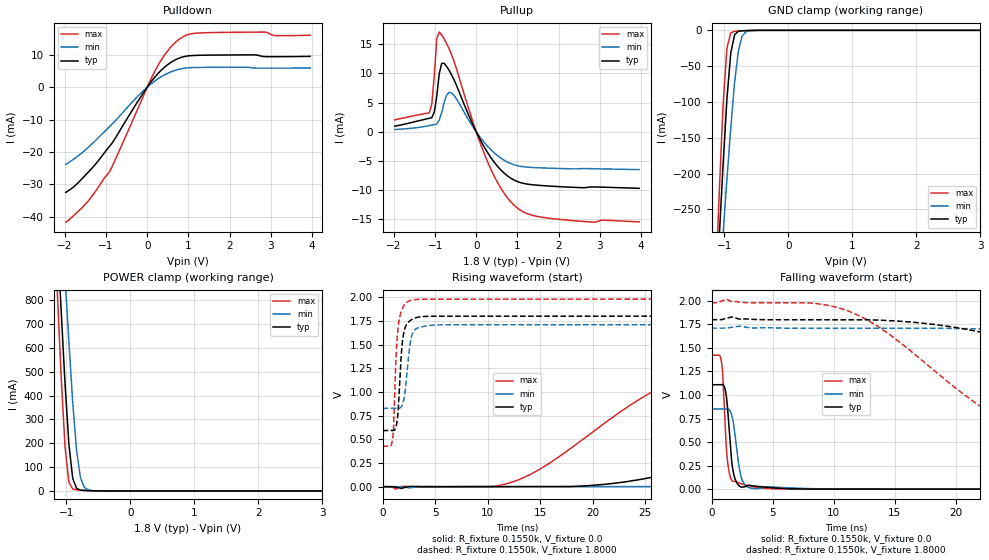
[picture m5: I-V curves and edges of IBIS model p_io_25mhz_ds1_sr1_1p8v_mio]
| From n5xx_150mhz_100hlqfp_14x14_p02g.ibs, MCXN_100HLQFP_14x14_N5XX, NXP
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[Model] p_io_25mhz_ds1_sr1_1p8v_mio
|   Model p_io_25mhz_ds1_sr1_1p8v_mio
| This model was characterised for following simulation conditions:
| External (pad) voltage:
|   - Typ: 1.8V,   - Min: 1.71V,   - Max: 1.98V
| Library cells for typ/min/max conditions are connected as defined below:
|  pad - External Pad
|  ipp_do_lv - Core Input
|  ipp_obe_lv - Output Buffer Enable
|  IOGC - NC
|  REFH3V3 - REFH3V3
|  REFL3V3 - REFL3V3
|  ZI - NC
|  abut_ncal_vddio[1] - vssio vddio vddio
|  abut_ncal_vddio[2] - vddio vddio vssio
|  abut_ncal_vddio[3] - vddio
|  abut_ncal_vddio[4] - vssio vddio vddio
|  abut_ncal_vddio[5] - vddio vddio vssio
|  abut_ncal_vddio[6] - vddio
|  abut_pcal_vddio[1] - vssio
|  abut_pcal_vddio[2] - vddio vssio vddio
|  abut_pcal_vddio[3] - vssio
|  abut_pcal_vddio[4] - vssio
|  abut_pcal_vddio[5] - vddio vssio vddio
|  abut_pcal_vddio[6] - vssio
|  ipp_do_1p8v - ipp_do_1p8v
|  ipp_dse_lv - vdd_lv
|  ipp_eftd_lv - NC
|  ipp_ina_mux_vddio - NC
|  ipp_ina_mux_vddio[0] - NC
|  ipp_ina_mux_vddio[1] - NC
|  ipp_ina_r0_vddio - NC
|  ipp_ina_r0a_vddio - NC
|  ipp_ina_r0b_vddio - NC
|  ipp_ina_r0c_vddio - NC
|  ipp_ina_r0d_vddio - NC
|  ipp_ina_r0e_vddio - NC
|  ipp_ina_r0f_vddio - NC
|  ipp_ina_r300_vddio - NC
|  ipp_ina_r300a_vddio - NC
|  ipp_ina_r300b_vddio - NC
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Model_type I/O
Polarity   Non-Inverting
Enable   Active-High
Vinl =   0.5400V
Vinh =   1.2600V
Vmeas =  0.9000V
Cref =   30.0000pF
Rref =   1.0000M
Vref =   1.8000V
C_comp   1.3069pF   1.2545pF   1.3693pF
|C_comp_pullup   0.5684pF   0.5978pF   0.5415pF
|C_comp_pulldown   0.6467pF   0.6779pF   0.6223pF
[Model Spec]
| variable   typ   min   max
Vinh   1.2600V   1.1970V   1.3860V
Vinl   0.5400V   0.5130V   0.5940V
[Temperature Range]   25.0000   0.1250k   -40.0000
[Voltage Range]   1.8000V   1.7100V   1.9800V
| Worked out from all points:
|   slope of the pulldown table from 0 to 0.27 V, typ, clamps not added: 62.4 ohm
|   slope of the pullup table from 0 to 0.27 V, typ, clamps not added: 77.5 ohm
|   GND clamp passes 1 mA (typ) near -0.75 V on its own axis
|   POWER clamp passes 1 mA (typ) near -0.63 V on its own axis
|   rising waveform, R_fixture 0.1550k, V_fixture 0.0: 20-80 % time 23.8ns typ, 44.7ns min, 12ns max; typ from 0 V to 1.11 V
|   rising waveform, R_fixture 0.1550k, V_fixture 1.8000: 20-80 % time 417ps typ, 512ps min, 381ps max; typ from 0.592 V to 1.8 V
|   falling waveform, R_fixture 0.1550k, V_fixture 0.0: 20-80 % time 432ps typ, 534ps min, 371ps max; typ from 1.11 V to 0 V
|   falling waveform, R_fixture 0.1550k, V_fixture 1.8000: 20-80 % time 19.3ns typ, 37.7ns min, 9.58ns max; typ from 1.8 V to 0.592 V
[Pulldown]
|Voltage   I(typ)   I(min)   I(max)
-1.98V    -32.47mA   -23.82mA   -41.66mA
-1.44V    -26.32mA   -18.64mA   -35.17mA
-900mV    -18mA      -11.95mA   -25.72mA
-180mV    -3.436mA   -2.171mA   -5.242mA
180mV     3.037mA    1.878mA    4.808mA
480mV     6.796mA    4.207mA    10.95mA
780mV     8.996mA    5.568mA    14.83mA
1.02V     9.701mA    6.008mA    16.34mA
1.38V     9.88mA     6.118mA    16.8mA
2.88V     9.438mA    5.883mA    17mA
3.12V     9.431mA    5.886mA    15.93mA
3.96V     9.527mA    5.94mA     16.05mA
[Pullup]
|Voltage   I(typ)   I(min)   I(max)
-1.98V    967.4uA    399.6uA    2.046mA
-1.14V    2.322mA    1.064mA    3.245mA
-1.08V    2.417mA    1.15mA     4.767mA
-1.02V    3.36mA     1.241mA    9.562mA
-960mV    6.043mA    1.333mA    15.9mA
-900mV    9.924mA    1.975mA    17.07mA
-780mV    11.72mA    5.036mA    15.9mA
-600mV    9.761mA    6.668mA    13.21mA
240mV     -3.146mA   -2.19mA    -4.535mA
900mV     -8.187mA   -5.593mA   -12.43mA
1.68V     -9.242mA   -6.203mA   -14.71mA
3.96V     -9.672mA   -6.474mA   -15.42mA
[GND_clamp]
|Voltage   I(typ)   I(min)   I(max)
-1.98V    -1.998A    -1.645A    -2.498A
-1.14V    -394mA     -441.4mA   -363.8mA
-1.08V    -288.3mA   -361.7mA   -226.5mA
-1.02V    -187.2mA   -283.6mA   -103.9mA
-960mV    -95.66mA   -207.9mA   -24.8mA
-900mV    -31.51mA   -136.2mA   -3.52mA
-840mV    -6.042mA   -72.18mA   -1.393mA
-780mV    -1.326mA   -27.91mA   -950.1uA
-720mV    -597.6uA   -7.636mA   -651.3uA
-660mV    -360.6uA   -1.814mA   -411.4uA
-420mV    -15.1uA    -32.81uA   -9.558uA
3.96V     0A         0A         0A
[POWER_clamp]
|Voltage   I(typ)   I(min)   I(max)
-1.98V    5.618A     5.349A     6.084A
-1.14V    1.071A     1.443A     829.5mA
-1.08V    754.2mA    1.168A     476.4mA
-1.02V    449mA      895.6mA    184.5mA
-960mV    195.8mA    625.5mA    36.73mA
-900mV    52.41mA    371.1mA    7.756mA
-840mV    10.72mA    170.2mA    4.398mA
-780mV    3.601mA    56.22mA    3.157mA
-720mV    2.062mA    15.03mA    2.179mA
-660mV    1.299mA    4.293mA    1.367mA
-360mV    5.029uA    27.47uA    1.319uA
3.96V     0A         0A         0A
[Ramp]
| variable   typ   min   max
dV/dt_r  0.6653/23.7529n   0.5079/44.7216n   0.8533/12.0054n
dV/dt_f  0.7248/19.2931n   0.5284/37.7240n   0.9320/9.5760n
R_load = 0.1550k
[Rising Waveform]
R_fixture= 0.1550k
V_fixture= 0.0
V_fixture_min= 0.0
V_fixture_max= 0.0
|time   V(typ)   V(min)   V(max)
0s        479.1pV    140.6nV    13.08pV
12.06ns   -29.43uV   -6.168uV   38.94mV
20.72ns   20.39mV    57.72uV    637.6mV
27.95ns   153.8mV    2.185mV    1.121V
41.83ns   590.6mV    71.17mV    1.346V
51.54ns   845.1mV    174.1mV    1.385V
61.62ns   966.4mV    306.4mV    1.404V
84.63ns   1.062V     594.8mV    1.418V
103.8ns   1.088V     716.8mV    1.421V
235ns     1.109V     846.5mV    1.422V
[Rising Waveform]
R_fixture= 0.1550k
V_fixture= 1.8000
V_fixture_min= 1.7100
V_fixture_max= 1.9800
|time   V(typ)   V(min)   V(max)
0s        591.9mV    826.9mV    426.6mV
967.4ps   591.6mV    826.9mV    511.4mV
1.069ns   592.4mV    826.9mV    674.8mV
1.342ns   663.2mV    826.9mV    1.488V
1.668ns   1.181V     830.8mV    1.806V
1.851ns   1.49V      857mV      1.871V
2.096ns   1.662V     962.5mV    1.922V
2.662ns   1.755V     1.536V     1.966V
3.301ns   1.787V     1.673V     1.976V
235ns     1.8V       1.71V      1.98V
[Falling Waveform]
R_fixture= 0.1550k
V_fixture= 0.0
V_fixture_min= 0.0
V_fixture_max= 0.0
|time   V(typ)   V(min)   V(max)
0s        1.109V     850.8mV    1.422V
803.8ps   1.11V      850.7mV    1.358V
920.3ps   1.11V      850.7mV    1.199V
1.239ns   958.7mV    853.6mV    388.3mV
1.586ns   381.7mV    812.7mV    109.8mV
1.934ns   104.1mV    563.4mV    83.46mV
2.272ns   33.66mV    222.5mV    63.14mV
2.579ns   22.27mV    75.81mV    50.55mV
4.791ns   16.79mV    24.39mV    5.652mV
235ns     96.44nV    1.938uV    11.99nV
[Falling Waveform]
R_fixture= 0.1550k
V_fixture= 1.8000
V_fixture_min= 1.7100
V_fixture_max= 1.9800
|time   V(typ)   V(min)   V(max)
0s        1.8V       1.71V      1.98V
10.68ns   1.8V       1.71V      1.915V
14.16ns   1.793V     1.71V      1.681V
24.07ns   1.608V     1.694V     724.5mV
35.2ns    1.158V     1.607V     506.4mV
42.57ns   884.8mV    1.511V     470.5mV
50.77ns   751.3mV    1.379V     450.8mV
68.52ns   653.9mV    1.096V     434.1mV
89.52ns   616.2mV    949.2mV    428.6mV
235ns     592mV      829.3mV    426.6mV
